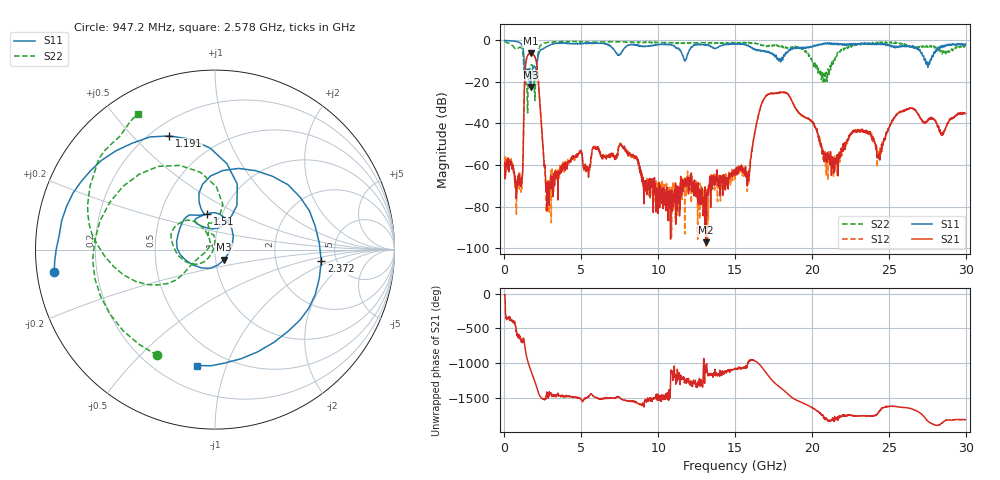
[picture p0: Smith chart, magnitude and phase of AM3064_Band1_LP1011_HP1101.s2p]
# Hz S DB R 50.0
!freq dBS11 angS11 dBS21 angS21 dBS12 angS12 dBS22 angS22
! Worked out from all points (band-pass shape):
!   1600 points, 10 MHz to 29.98 GHz, reference 50 ohm
!   highest |S21| = -6.21 dB at 1.697 GHz (marker M1); lowest = -97.2 dB at 13.09 GHz (marker M2)
!   |S21| within 3 dB of the highest: 1.426 GHz to 2.041 GHz (614.6 MHz wide, 35.5 % of centre)
!   lowest |S11| = -22.4 dB at 1.697 GHz (marker M3), VSWR 1.16, Z = 54.9 - j6.26 ohm
!   |S11| at or under -10 dB: 1.277 GHz to 2.143 GHz (866.2 MHz wide, 50.7 % of centre); 17.9525 GHz to 17.9865 GHz (34 MHz wide, 0.189 % of centre); 27.4 GHz to 27.68 GHz (283.1 MHz wide, 1.03 % of centre)
!   |S22| runs from -35.0 to -0.3 dB; largest |S21 - S12| = 0.006
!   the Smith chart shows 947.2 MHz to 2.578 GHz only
!   S11 on the Smith chart (normalised r, x): 947.2 MHz: 0.05, -0.07; 1.191 GHz: 0.27, +0.64; 1.51 GHz: 0.85, +0.35; 2.372 GHz: 3.79, -0.75; 2.578 GHz: 0.35, -0.80
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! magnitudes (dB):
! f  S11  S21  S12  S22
! 10 MHz  0.0  -58.6  -55.7  -0.3
! 947.2 MHz  -0.9  -66.8  -67.8  -3.5
! 1.191 GHz  -3.3  -62.5  -61.0  -5.9
! 1.51 GHz  -13.9  -7.2  -7.2  -35.0
! 1.697 GHz  -22.4  -6.2  -6.2  -12.5
! 2.072 GHz  -13.7  -10.2  -10.2  -13.8
! 2.372 GHz  -4.5  -37.1  -37.1  -2.1
! 2.578 GHz  -3.7  -60.5  -57.1  -1.2
! 2.822 GHz  -2.7  -68.9  -76.2  -1.0
! 5.015 GHz  -1.5  -54.7  -54.6  -0.7
! 7.62 GHz  -5.6  -50.2  -50.1  -0.7
! 10 GHz  -2.0  -72.5  -69.8  -1.0
! 13.09 GHz  -2.1  -97.2  -75.9  -1.0
! 15 GHz  -1.8  -65.0  -62.8  -1.4
! 15.83 GHz  -2.7  -64.3  -65.9  -1.4
! 17.14 GHz  -5.6  -25.9  -25.9  -2.8
! 19.99 GHz  -3.2  -39.1  -39.3  -9.3
! 21.49 GHz  -1.3  -58.0  -55.4  -9.6
! 22.69 GHz  -1.5  -43.8  -43.7  -2.8
! 24.36 GHz  -1.7  -56.2  -55.0  -1.5
! 25 GHz  -2.0  -42.3  -42.6  -1.0
! 29.98 GHz  -1.7  -35.2  -35.0  -3.0
